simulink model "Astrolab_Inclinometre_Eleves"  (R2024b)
settings: Solver=FixedStepDiscrete  StartTime=0.0  StopTime=inf  FixedStep=0.5e-5  RelTol=1e-3  EnableMultiTasking=on
undefined symbols (not defined in the file): daq, Dev1, ni, USB
libraries: daqlib x3, dspstat3 x2

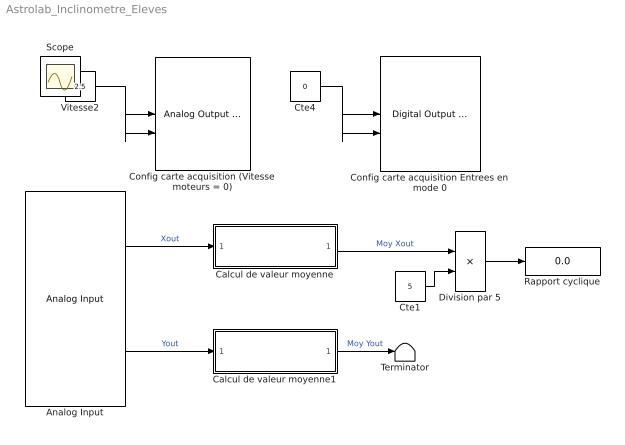
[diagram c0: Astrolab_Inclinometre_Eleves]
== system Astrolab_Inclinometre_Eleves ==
  Analog Input : daqlib/Analog Input  DeviceMenu=(none)  Device=ni Dev1 (USB-6009OEM2)  ObjConstructor=daq.createSession('ni')  NChannelsSelected=2  Channels=0$ai0$$Dev1$1$8$2$1$#0$ai1$$Dev1$1$8$2$1$#1$ai2$$Dev1$1$7$1$1$#1$ai3$$Dev1$1$7$1$1$#0$ai4$$Dev1$1$7$1$1$#0$ai5$$Dev1$1$7$1$1$#0$ai6$$Dev1$1$7$1$1$#0$ai7$$Dev1$1$7$1$1$#  NPorts=1 per channel  SampleRate=2000  ActualRate=2000  ScansPerTrigger=100  OutputTimestamp=off  AcqMode=0  NumFrameBuffer=100  OutputTriggertime=off
  Calcul de valeur moyenne : Subsystem
  Calcul de valeur moyenne1 : Subsystem
  Config carte acquisition (Vitesse moteurs = 0) : daqlib/Analog Output (Single Sample)  DeviceMenu=(none)  Device=ni Dev1 (USB-6009OEM2)  ObjConstructor=daq.createSession('ni')  NChannelsSelected=2  Channels=1$ao0$$Dev1$1$1$N/A$#1$ao1$$Dev1$1$1$N/A$#  NPorts=1 per channel  BlockSampleTime=1
  Config carte acquisition Entrees en mode 0 : daqlib/Digital Output (Single Sample)  DeviceMenu=(none)  Device=ni Dev1 (USB-6009OEM2)  ObjConstructor=daq.createSession('ni')  BlockSampleTime=1  IsDigitalInput=off  NLinesSelected=2  Lines=1$port0/line0$$Dev1$#1$port0/line1$$Dev1$#0$port0/line2$$Dev1$#0$port0/line3$$Dev1$#0$port0/line4$$Dev1$#0$port0/line5$$Dev1$#0$port0/line6$$Dev1$#0$port0/line7$$Dev1$#0$port1/line0$$Dev1$#0$port1/line1$$Dev1$#0$port1/line2$$Dev1$#0$port1/line3$$Dev1$#  NPorts=1 per line
  Cte1 : Constant  Value=5
  Cte4 : Constant  Value=0  OutDataTypeStr=boolean
  Division par 5 : Product  Inputs=*/
  Rapport cyclique : Display
  Terminator : Terminator
  Vitesse2 : Constant  Value=2.5
  Scope : Scope
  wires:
  Vitesse2/1 -> Config carte acquisition (Vitesse moteurs = 0)/2, Config carte acquisition (Vitesse moteurs = 0)/1
  Cte4/1 -> Config carte acquisition Entrees en mode 0/2, Config carte acquisition Entrees en mode 0/1
  Analog Input/2 -> Calcul de valeur moyenne1/1(Xout)  "Yout"
  Calcul de valeur moyenne1/1(Out1) -> Terminator/1  "Moy Yout"
  Cte1/1 -> Division par 5/2
  Division par 5/1 -> Rapport cyclique/1
  Analog Input/1 -> Calcul de valeur moyenne/1(Xout)  "Xout"
  Calcul de valeur moyenne/1(Out1) -> Division par 5/1  "Moy Xout"

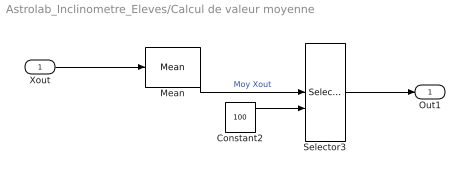
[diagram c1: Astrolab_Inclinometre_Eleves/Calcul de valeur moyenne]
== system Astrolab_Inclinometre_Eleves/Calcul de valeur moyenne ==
  Xout : Inport
  Constant2 : Constant  Value=100
  Mean : dspstat3/Mean  run=on  reset_popup=None  InputProcessing=Columns as channels (frame based)  directionMode=Each column  dimension=1  roiEnable=off  roiType=Rectangles  roiPortion=Entire ROI  roiOutput=Individual statistics for each ROI  roiFlag=off  outputDataTypeStr=Inherit: Same as accumulator  outputLastDataTypeStr=Inherit: Same as accumulator  outputMin=[]  outputMax=[]  roundingMode=Floor  overflowMode=off
  Selector3 : Selector  InputPortWidth=100  IndexOptions=Index vector (port)  Indices=[1 3]  OutputSizes=1
  Out1 : Outport  VectorParamsAs1DForOutWhenUnconnected=off
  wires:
  Mean/1 -> Selector3/1  "Moy Xout"
  Xout/1 -> Mean/1
  Selector3/1 -> Out1/1
  Constant2/1 -> Selector3/2

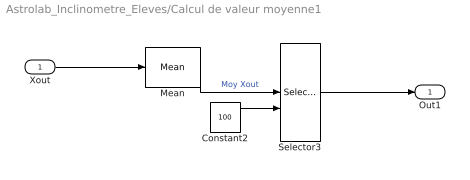
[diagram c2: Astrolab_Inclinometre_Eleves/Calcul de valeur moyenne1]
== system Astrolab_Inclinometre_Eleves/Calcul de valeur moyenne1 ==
  Xout : Inport
  Constant2 : Constant  Value=100
  Mean : dspstat3/Mean  run=on  reset_popup=None  InputProcessing=Columns as channels (frame based)  directionMode=Each column  dimension=1  roiEnable=off  roiType=Rectangles  roiPortion=Entire ROI  roiOutput=Individual statistics for each ROI  roiFlag=off  outputDataTypeStr=Inherit: Same as accumulator  outputLastDataTypeStr=Inherit: Same as accumulator  outputMin=[]  outputMax=[]  roundingMode=Floor  overflowMode=off
  Selector3 : Selector  InputPortWidth=100  IndexOptions=Index vector (port)  Indices=[1 3]  OutputSizes=1
  Out1 : Outport  VectorParamsAs1DForOutWhenUnconnected=off
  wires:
  Constant2/1 -> Selector3/2
  Selector3/1 -> Out1/1
  Xout/1 -> Mean/1
  Mean/1 -> Selector3/1  "Moy Xout"
